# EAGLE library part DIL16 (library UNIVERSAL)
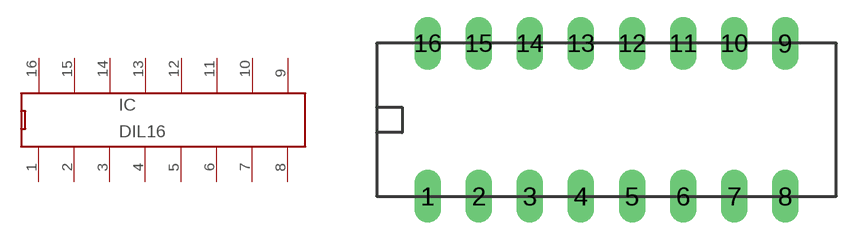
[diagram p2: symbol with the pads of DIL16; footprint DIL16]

Designator prefix IC

## DIL16  [DIL16]
1  P$1
2  P$2
3  P$3
4  P$4
5  P$5
6  P$6
7  P$7
8  P$8
9  P$9
10  P$10
11  P$11
12  P$12
13  P$13
14  P$14
15  P$15
16  P$16

## Footprint DIL16 (pad centres in mm)
drill 0.813 pad 1.27 long: 1 0,1.27; 2 2.54,1.27; 3 5.08,1.27; 4 7.62,1.27; 5 10.16,1.27; 6 12.7,1.27; 7 15.24,1.27; 8 17.78,1.27; 9 17.78,8.89; 10 15.24,8.89; 11 12.7,8.89; 12 10.16,8.89; 13 7.62,8.89; 14 5.08,8.89; 15 2.54,8.89; 16 0,8.89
